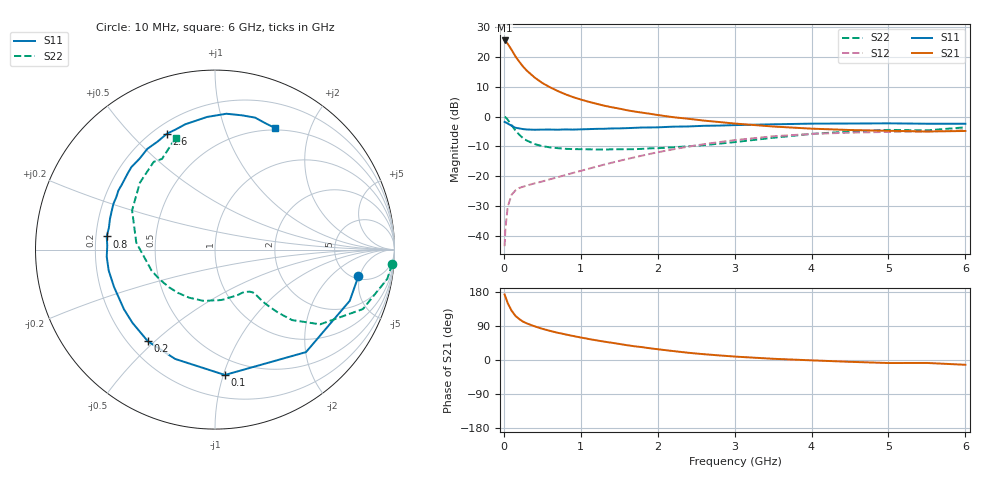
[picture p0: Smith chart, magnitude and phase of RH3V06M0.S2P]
! SIEMENS Small Signal Semiconductors
! BFR106
! Si NPN RF Bipolar Junction Transistor in SOT23
! VCE = 3 V  IC = 6 mA
! Common Emitter S-Parameters:  August  1996
# GHz  S  MA  R  50
!  f  S11  S21  S12  S22
! GHz  MAG  ANG  MAG  ANG  MAG  ANG  MAG  ANG
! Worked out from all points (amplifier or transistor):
!   36 points, 10 MHz to 6 GHz, reference 50 ohm
!   highest |S21| = 25.5 dB at 10 MHz (marker M1)
!   |S21| within 3 dB of that: start of sweep to 97.36 MHz
!   unconditionally stable (mu >= 1): 593.6 MHz to 2.089 GHz; 4.709 GHz to end of sweep
!   at 250 MHz: K = 0.56, MSG = 20.1 dB, |S12| = -23.5 dB
!   at 1.4 GHz: K = 1.13, MAG = 7.1 dB, |S12| = -15.5 dB
!   at 6 GHz: K = 1.02, MAG = -1.0 dB, |S12| = -4.6 dB
!   S11 on the Smith chart (normalised r, x): 10 MHz: 5.50, -4.75; 100 MHz: 0.37, -1.01; 200 MHz: 0.28, -0.48; 800 MHz: 0.24, +0.06; 2.6 GHz: 0.25, +0.64; 6 GHz: 0.47, +1.50
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0.01  0.8128 -10.4  18.85 172.9  0.0067 84.7  0.9897 -4.7
0.02  0.8031 -20.8  18.5 167.4  0.0129 80.4  0.974 -9.6
0.05  0.7637 -48.4  16.59 150.3  0.0304 66.3  0.8883 -21.9
0.1  0.7006 -85.5  13.19 130.4  0.0487 52.6  0.7187 -35.4
0.15  0.6484 -110.0  10.24 116.6  0.0575 43.9  0.5825 -42.4
0.2  0.6331 -126.2  8.316 108.1  0.0634 41.1  0.497 -45.0
0.25  0.6148 -138.4  6.883 101.2  0.0666 39.3  0.4324 -46.5
0.3  0.6064 -146.8  5.85 96.5  0.0697 39.6  0.3947 -47.4
0.4  0.5999 -159.7  4.515 88.9  0.0757 41.5  0.3452 -47.8
0.5  0.6037 -168.9  3.651 82.4  0.0814 44.2  0.3185 -48.5
0.6  0.6045 -176.2  3.095 76.9  0.0887 46.9  0.3038 -50.5
0.8  0.6078 173.1  2.36 67.6  0.1045 51.7  0.2872 -55.6
0.9  0.6036 168.3  2.115 63.4  0.1134 53.8  0.284 -58.2
1.1  0.6145 159.4  1.772 55.6  0.1329 57.0  0.2817 -66.2
1.3  0.6228 152.0  1.524 48.6  0.1557 58.9  0.279 -74.1
1.6  0.6385 141.9  1.274 39.1  0.1934 59.5  0.283 -87.9
2.2  0.6761 123.9  0.975 23.6  0.2818 55.3  0.3044 -118.5
2.6  0.6989 112.6  0.855 15.3  0.3431 49.7  0.331 -140.6
3.5  0.7404 93.4  0.68 3.2  0.4661 33.7  0.4404 174.9
4.5  0.7631 78.6  0.594 -4.8  0.5363 15.2  0.5604 138.3
5.5  0.7571 67.6  0.561 -7.8  0.5617 3.9  0.5853 120.3
6  0.7559 63.8  0.572 -12.6  0.5877 -3.7  0.6592 109.5
